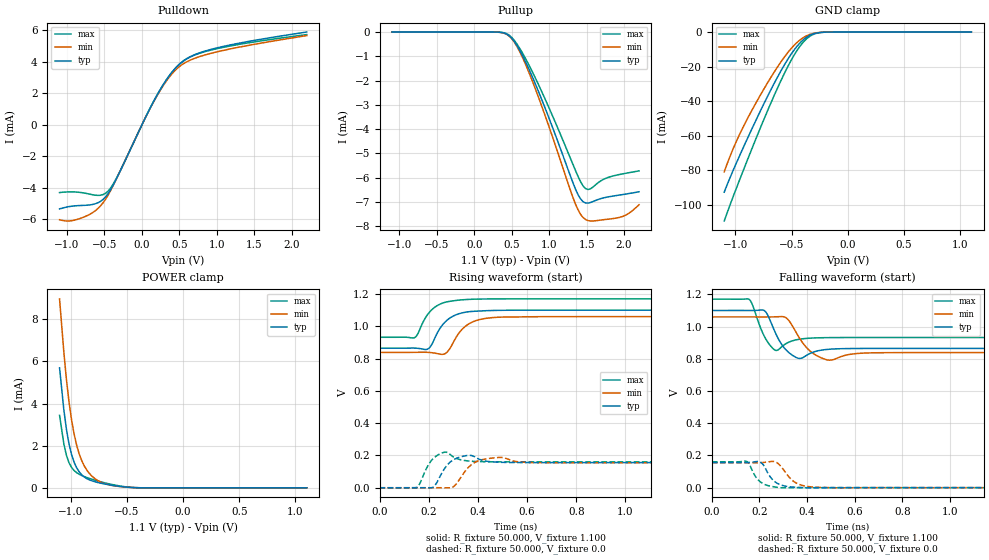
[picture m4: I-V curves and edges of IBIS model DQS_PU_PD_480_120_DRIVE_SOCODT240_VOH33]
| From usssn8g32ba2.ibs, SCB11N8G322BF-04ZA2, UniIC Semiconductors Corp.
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|   Model DQS_PU_PD_480_120_DRIVE_SOCODT240_VOH33
[Model] DQS_PU_PD_480_120_DRIVE_SOCODT240_VOH33
Model_type I/O
Polarity   Inverting
Vinl =  98.000mV
Vinh =  0.268V
Vmeas =  0.183V
Rref =  50.000
Vref =  0.183V
C_comp   1.020pF   1.010pF   1.030pF
[Model Spec]
Vinh   0.268V   0.262V   0.280V
Vinl   98.000mV   92.000mV   0.110V
Vmeas   0.183V   0.177V   0.195V
Vref   0.183V   0.177V   0.195V
Rref   50.000   NA   NA
[Temperature Range]   25.000   0.105k   -40.000
[Voltage Range]   1.100V   1.060V   1.170V
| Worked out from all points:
|   slope of the pulldown table from 0 to 0.165 V, typ, clamps not added: 105 ohm
|   GND clamp passes 1 mA (typ) near -0.30 V on its own axis
|   POWER clamp passes 1 mA (typ) near -0.95 V on its own axis
|   rising waveform, R_fixture 50.000, V_fixture 1.100: 20-80 % time 67.3ps typ, 70.1ps min, 65.3ps max; typ from 0.864 V to 1.1 V
|   rising waveform, R_fixture 50.000, V_fixture 0.0: 20-80 % time 34.8ps typ, 44.3ps min, 28.1ps max; typ from 0 V to 0.156 V
|   falling waveform, R_fixture 50.000, V_fixture 1.100: 20-80 % time 43.5ps typ, 56.6ps min, 34.2ps max; typ from 1.1 V to 0.864 V
|   falling waveform, R_fixture 50.000, V_fixture 0.0: 20-80 % time 47.2ps typ, 57.4ps min, 44.1ps max; typ from 0.156 V to 0 V
[Pulldown]
|Voltage   I(typ)   I(min)   I(max)
-1.1V     -5.34mA    -6.026mA   -4.302mA
-930mV    -5.164mA   -6.082mA   -4.26mA
-726mV    -5.101mA   -5.754mA   -4.373mA
-556mV    -4.87mA    -5.165mA   -4.475mA
-454mV    -4.386mA   -4.479mA   -4.222mA
-318mV    -3.209mA   -3.211mA   -3.18mA
192mV     1.799mA    1.766mA    1.806mA
362mV     3.096mA    3.011mA    3.096mA
532mV     3.983mA    3.811mA    3.973mA
702mV     4.448mA    4.219mA    4.427mA
1.008V    4.891mA    4.64mA     4.842mA
2.2V      5.891mA    5.665mA    5.73mA
[Pullup]
|Voltage   I(typ)   I(min)   I(max)
-1.1V     500pA      5.412nA    0A
432mV     -84.42uA   -95.4uA    -65.89uA
568mV     -546.4uA   -585.3uA   -487.9uA
704mV     -1.354mA   -1.473mA   -1.207mA
942mV     -3.104mA   -3.412mA   -2.737mA
1.316V    -6.198mA   -6.807mA   -5.446mA
1.418V    -6.872mA   -7.507mA   -6.161mA
1.52V     -7.049mA   -7.771mA   -6.489mA
1.724V    -6.835mA   -7.734mA   -6.072mA
1.894V    -6.739mA   -7.667mA   -5.9mA
2.03V     -6.672mA   -7.532mA   -5.816mA
2.2V      -6.582mA   -7.117mA   -5.721mA
[GND_clamp]
|Voltage   I(typ)   I(min)   I(max)
-1.1V     -92.78mA   -81.05mA   -109.5mA
-1.031V   -81.73mA   -69.22mA   -97.17mA
-939mV    -68.18mA   -56.02mA   -81.64mA
-824mV    -52mA      -41.83mA   -62.83mA
-686mV    -33.62mA   -26.41mA   -41.32mA
-571mV    -19.76mA   -15.06mA   -24.85mA
-479mV    -10.5mA    -7.76mA    -13.5mA
-410mV    -5.313mA   -3.84mA    -6.916mA
-341mV    -2.007mA   -1.45mA    -2.59mA
-272mV    -506.9uA   -403.5uA   -609.8uA
-180mV    -45.65uA   -51.35uA   -43.55uA
1.1V      0A         0A         0A
[POWER_clamp]
|Voltage   I(typ)   I(min)   I(max)
-1.1V     5.691mA    8.967mA    3.44mA
-1.062V   3.709mA    6.444mA    2.092mA
-1.039V   2.781mA    5.152mA    1.546mA
-1.016V   2.086mA    4.085mA    1.193mA
-970mV    1.21mA     2.539mA    818.5uA
-947mV    943.7uA    2.005mA    716.7uA
-901mV    610.1uA    1.27mA     581.3uA
-855mV    430.7uA    824.1uA    484.6uA
-786mV    289.9uA    439.4uA    366uA
-671mV    155.9uA    155.9uA    203.6uA
-441mV    13.2uA     12.79uA    15.03uA
1.1V      0A         0A         0A
[Ramp]
| variable   typ   min   max
dV/dt_r   93.600m/34.847p   92.825m/44.278p   96.210m/28.119p
dV/dt_f   0.141/43.472p   0.133/56.639p   0.143/34.237p
R_load = 50.000
[Rising Waveform]
R_fixture= 50.000
V_fixture= 1.100
V_fixture_min= 1.060
V_fixture_max= 1.170
|time   V(typ)   V(min)   V(max)
0s        864.4mV    838.5mV    932.1mV
143ps     864.9mV    838.8mV    930.3mV
195ps     858.5mV    838.9mV    1.072V
260ps     1.016V     827mV      1.146V
281ps     1.046V     850.9mV    1.153V
302ps     1.065V     905.9mV    1.158V
358ps     1.089V     1.01V      1.166V
421ps     1.096V     1.046V     1.169V
513ps     1.099V     1.057V     1.17V
3ns       1.1V       1.06V      1.17V
[Rising Waveform]
R_fixture= 50.000
V_fixture= 0.0
V_fixture_min= 0.0
V_fixture_max= 0.0
|time   V(typ)   V(min)   V(max)
0s        4.355uV    15.89uV    1.03uV
153ps     74.34uV    33.99uV    3.815mV
220ps     6.161mV    156.2uV    183.2mV
269ps     128.3mV    -477.5uV   220.6mV
307ps     178.3mV    14.88mV    185.6mV
359ps     200.5mV    121.9mV    166.2mV
406ps     176.2mV    169mV      161.9mV
486ps     157.9mV    187.7mV    160.5mV
641ps     156mV      155.3mV    160.3mV
3ns       156mV      154.7mV    160.3mV
[Falling Waveform]
R_fixture= 50.000
V_fixture= 1.100
V_fixture_min= 1.060
V_fixture_max= 1.170
|time   V(typ)   V(min)   V(max)
0s        1.1V       1.06V      1.17V
157ps     1.1V       1.06V      1.168V
222ps     1.097V     1.06V      934.8mV
269ps     954.3mV    1.061V     852.1mV
314ps     851.5mV    1.052V     896.3mV
359ps     804.9mV    950.9mV    919.1mV
414ps     834.3mV    846.1mV    928.2mV
492ps     859.1mV    791.5mV    931.4mV
685ps     864.3mV    837.3mV    932.1mV
3ns       864.4mV    838.5mV    932.1mV
[Falling Waveform]
R_fixture= 50.000
V_fixture= 0.0
V_fixture_min= 0.0
V_fixture_max= 0.0
|time   V(typ)   V(min)   V(max)
0s        156mV      154.7mV    160.3mV
146ps     155.8mV    154.5mV    162.8mV
200ps     160.7mV    154.8mV    40.46mV
216ps     141.6mV    156.3mV    23.92mV
260ps     42.69mV    162.3mV    5.488mV
292ps     15.89mV    128mV      -493.3uV
325ps     5.772mV    64.19mV    -412.7uV
351ps     2.612mV    31.47mV    -181.2uV
446ps     -480.7uV   2.154mV    -7.656uV
3ns       4.229uV    15.82uV    788.9nV
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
